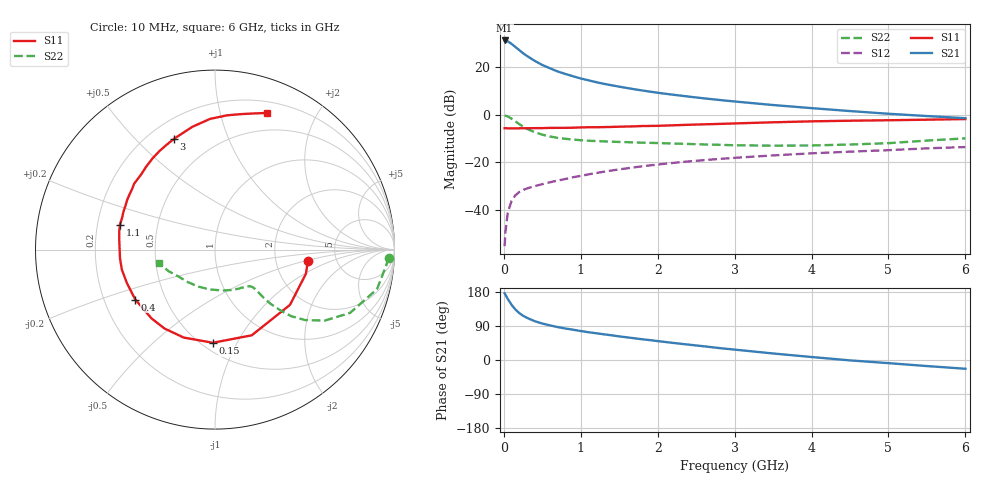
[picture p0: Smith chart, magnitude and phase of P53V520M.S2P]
! SIEMENS Small Signal Semiconductors
! BFP183
! Si NPN RF Bipolar Junction Transistor in SOT143
! VCE = 3.5 V  IC = 20 mA
! Common Emitter S-Parameters:  March  1996
# GHz  S  MA  R  50
!  f  S11  S21  S12  S22
! GHz  MAG  ANG  MAG  ANG  MAG  ANG  MAG  ANG
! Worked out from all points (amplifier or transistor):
!   36 points, 10 MHz to 6 GHz, reference 50 ohm
!   highest |S21| = 31.4 dB at 10 MHz (marker M1)
!   |S21| within 3 dB of that: start of sweep to 160 MHz
!   unconditionally stable (mu >= 1): 801.6 MHz to 5.578 GHz
!   at 250 MHz: K = 0.48, MSG = 28.9 dB, |S12| = -31.7 dB
!   at 1.4 GHz: K = 1.13, MAG = 15.8 dB, |S12| = -23.5 dB
!   at 6 GHz: K = 0.94, MSG = 6.1 dB, |S12| = -13.6 dB
!   S11 on the Smith chart (normalised r, x): 10 MHz: 3.07, -0.55; 150 MHz: 0.56, -0.80; 400 MHz: 0.34, -0.26; 1.1 GHz: 0.30, +0.12; 3 GHz: 0.30, +0.65; 6 GHz: 0.31, +1.40
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0.01  0.5213 -7.2  37.02 176.1  0.0017 80.9  0.9685 -2.7
0.02  0.5242 -14.8  36.82 172.6  0.0033 86.6  0.9571 -5.5
0.05  0.5191 -36.4  35.55 161.4  0.0085 79.9  0.9293 -13.7
0.1  0.5195 -66.8  31.38 145.7  0.0153 65.6  0.8313 -25.1
0.15  0.5192 -91.3  27.02 133.3  0.0201 58.1  0.7283 -32.9
0.2  0.5201 -109.5  23.2 123.9  0.0235 53.4  0.6379 -38.0
0.25  0.5221 -122.5  19.95 116.7  0.026 50.8  0.565 -41.1
0.3  0.5215 -132.7  17.46 111.3  0.028 49.7  0.5071 -42.7
0.4  0.5241 -147.9  13.79 102.5  0.0313 48.9  0.4312 -44.3
0.5  0.5251 -159.2  11.25 96.2  0.0345 48.2  0.3815 -44.7
0.6  0.5307 -167.9  9.585 91.2  0.0378 50.2  0.3491 -44.6
0.7  0.5315 -174.5  8.212 86.9  0.0412 50.6  0.3269 -44.5
0.9  0.5356 174.7  6.509 79.9  0.0484 52.3  0.3009 -44.7
1.1  0.5476 165.3  5.344 73.3  0.0556 53.1  0.2844 -46.0
1.5  0.5619 150.7  3.926 62.3  0.0708 52.7  0.2681 -50.3
1.8  0.5811 140.9  3.265 54.7  0.0819 51.4  0.2582 -55.4
2.2  0.6012 129.4  2.656 45.1  0.0968 48.6  0.2481 -63.1
3  0.6586 110.2  1.912 27.4  0.1239 42.1  0.2282 -83.2
3.5  0.6959 100.4  1.61 17.2  0.1395 37.7  0.2239 -97.9
4.5  0.7513 84.8  1.201 -1.0  0.1673 28.8  0.2364 -130.2
5.5  0.7897 73.9  0.943 -16.0  0.1966 20.9  0.2865 -155.5
6  0.8144 69.2  0.849 -23.1  0.2092 16.4  0.3193 -166.3
